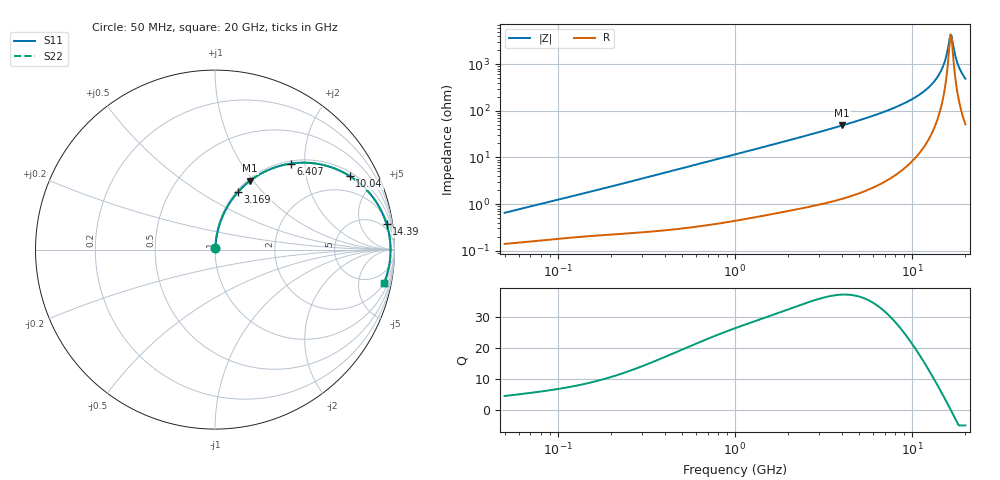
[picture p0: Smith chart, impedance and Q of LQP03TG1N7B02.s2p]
!Murata Part Number: LQP03TG1N7B02
!These Parameters are Measured in Series Mode Connection
!  o--[Z]--o
!Port1  Port2
!  o-------o
!Freq. Start=50[MHz] Stop=20[GHz], 401[Steps]
# Hz S RI R 50
!Freq.(Hz) S11(Real) S11(Imag) S21(Real) S21(Imag) S12(Real) S12(Imag) S22(Real) S22(Imag)
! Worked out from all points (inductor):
!   401 points, 50 MHz to 20 GHz, reference 50 ohm
!   read as one part in series: L = 1.99 nH near 51.52 MHz
!   highest Q = 37.4 at 4.027 GHz (marker M1), where L = 1.91 nH
!   self-resonance near 16.46 GHz
!   S11 on the Smith chart (normalised r, x): 50 MHz: 1.00, +0.01; 3.169 GHz: 1.02, +0.74; 6.407 GHz: 1.05, +1.70; 10.04 GHz: 1.17, +3.57; 14.39 GHz: 3, +13; 20 GHz: 2.02, -9.66
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5e7  0.00143 0.00631  0.9986 -0.00631  0.9986 -0.00631  0.00143 0.00631
1.364002e8  0.00225 0.0163  0.9978 -0.0163  0.9978 -0.0163  0.00225 0.0163
3.721004e8  0.00451 0.0431  0.9955 -0.0431  0.9955 -0.0431  0.00451 0.0431
1e9  0.0173 0.1129  0.9827 -0.1129  0.9827 -0.1129  0.0173 0.1129
2.728004e9  0.0982 0.2838  0.9018 -0.2838  0.9018 -0.2838  0.0982 0.2838
3.168813e9  0.1282 0.3209  0.8718 -0.3209  0.8718 -0.3209  0.1282 0.3209
4.026975e9  0.1956 0.3835  0.8044 -0.3835  0.8044 -0.3835  0.1956 0.3835
6.406762e9  0.4207 0.4791  0.5793 -0.4791  0.5793 -0.4791  0.4207 0.4791
7.442007e9  0.5233 0.4833  0.4767 -0.4833  0.4767 -0.4833  0.5233 0.4833
1.004137e10  0.7511 0.4095  0.2489 -0.4095  0.2489 -0.4095  0.7511 0.4095
1.238412e10  0.8915 0.2752  0.1085 -0.2752  0.1085 -0.2752  0.8915 0.2752
1.354865e10  0.9352 0.1979  0.0648 -0.1979  0.0648 -0.1979  0.9352 0.1979
1.438523e10  0.9565 0.1414  0.0435 -0.1414  0.0435 -0.1414  0.9565 0.1414
1.527346e10  0.9708 0.0821  0.0292 -0.0821  0.0292 -0.0821  0.9708 0.0821
1.621653e10  0.9776 0.021  0.0224 -0.021  0.0224 -0.021  0.9776 0.021
1.646126e10  0.9781 0.00561  0.0219 -0.00561  0.0219 -0.00561  0.9781 0.00561
1.670968e10  0.9781 -0.00979  0.0219 0.00979  0.0219 0.00979  0.9781 -0.00979
1.696185e10  0.9776 -0.0252  0.0224 0.0252  0.0224 0.0252  0.9776 -0.0252
1.774144e10  0.9732 -0.0711  0.0268 0.0711  0.0268 0.0711  0.9732 -0.0711
1.828096e10  0.9679 -0.1014  0.0321 0.1014  0.0321 0.1014  0.9679 -0.1014
1.912117e10  0.9565 -0.1458  0.0435 0.1458  0.0435 0.1458  0.9565 -0.1458
2e10  0.9411 -0.1886  0.0589 0.1886  0.0589 0.1886  0.9411 -0.1886
